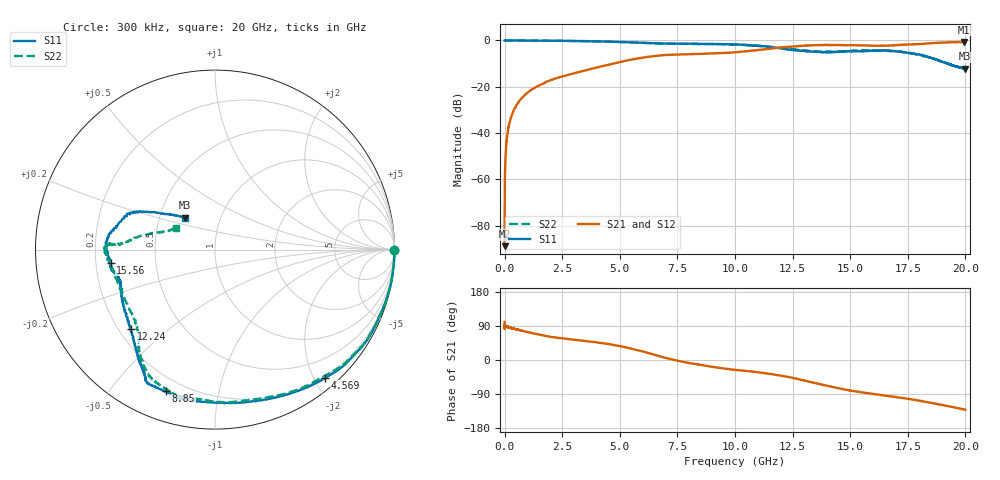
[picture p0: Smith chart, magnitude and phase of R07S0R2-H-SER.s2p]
!{R07S0R2}
!Johanson Technology Inc.
!www.johansontechnology.com
!Test Board Conditions:
!Substrate Type  RO4350B
!Substrate Thickness  10 mil
!Substrate Dk  3.66
!TL Type: GCPW
!TL Trace Width  21 mil
!TL Gap  20 mil
!Electrode orientation  Horizontal
!DUT TOPOLOGY	SERIES
!Mounting Pad LxW  16x21 mil
! Created Fri Feb  5 23:01:04 2021
# hz S ma R 50
! 2 Port Network Data from SP1.SP block
! freq  magS11  angS11  magS21  angS21  magS12  angS12  magS22  angS22
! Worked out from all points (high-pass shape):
!   20001 points, 300 kHz to 20 GHz, reference 50 ohm
!   highest |S21| = -0.64 dB at 19.95 GHz (marker M1); lowest = -88.9 dB at 300 kHz (marker M2)
!   |S21| within 3 dB of the highest: 11.44742 GHz to 11.44906 GHz (1.636 MHz wide, 0.0143 % of centre); 11.45 GHz to end of sweep
!   lowest |S11| = -12.2 dB at 19.99 GHz (marker M3), VSWR 1.65, Z = 33.6 + j12.8 ohm
!   |S11| at or under -10 dB: 19.23785 GHz to 19.23882 GHz (969.7 kHz wide, 0.00504 % of centre); 19.24 GHz to end of sweep
!   |S22| runs from -12.1 to 0.0 dB; largest |S21 - S12| = 0.021
!   S11 on the Smith chart (normalised r, x): 300 kHz: open; 4.569 GHz: 0.17, -2.16; 8.85 GHz: 0.13, -0.70; 12.24 GHz: 0.25, -0.38; 15.56 GHz: 0.26, -0.06; 20 GHz: 0.67, +0.26
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300000  0.9981 -0.2  3.606e-05 100.5  4.541e-05 42.4  1 -0.2
1.043e8  0.9988 -1.8  0.008254 88.1  0.008313 87.6  1 -1.7
1.513e8  0.9994 -2.6  0.01188 86.5  0.01204 86.9  0.9999 -2.6
2.993e8  0.9995 -5.2  0.02362 84.1  0.02365 84.0  0.9991 -5.1
5.513e8  0.9989 -9.3  0.04275 80.1  0.0428 80.4  0.9982 -9.2
9.373e8  0.9955 -15.1  0.07077 74.4  0.07081 74.3  0.9963 -15.1
1.4693e9  0.988 -22.3  0.1048 67.3  0.1053 67.3  0.9882 -22.1
3.3343e9  0.9699 -39.2  0.2143 51.2  0.2154 51.2  0.9687 -37.5
4.5693e9  0.9427 -49.4  0.3033 41.6  0.3049 41.5  0.9424 -46.4
6.6673e9  0.8662 -78.9  0.4696 10.9  0.471 11.2  0.8587 -78.0
7.9713e9  0.8515 -100.5  0.5031 -7.5  0.5082 -7.3  0.841 -93.8
8.8503e9  0.8358 -109.1  0.5204 -16.4  0.5198 -16.6  0.8399 -103.4
1.00003e10  0.8241 -117.9  0.5558 -26.0  0.5586 -25.9  0.8112 -112.8
1.13483e10  0.7423 -124.9  0.6494 -35.3  0.6548 -35.3  0.7391 -123.4
1.22423e10  0.6436 -136.7  0.7207 -43.9  0.7151 -44.6  0.671 -129.1
1.33343e10  0.572 -155.0  0.7841 -58.9  0.7783 -59.1  0.5885 -141.5
1.55613e10  0.5863 -172.9  0.7796 -85.8  0.7708 -85.6  0.6164 -178.7
1.66673e10  0.6029 174.3  0.7806 -95.4  0.7834 -94.5  0.5948 176.8
1.79293e10  0.5014 156.0  0.8339 -106.7  0.8389 -106.5  0.4923 174.9
1.99543e10  0.248 133.8  0.9289 -130.6  0.9299 -130.4  0.2527 150.9
1.99893e10  0.2454 133.3  0.9265 -131.2  0.9297 -130.9  0.2509 150.6
2e10  0.2465 133.2  0.9269 -131.2  0.932 -131.1  0.2496 150.6
